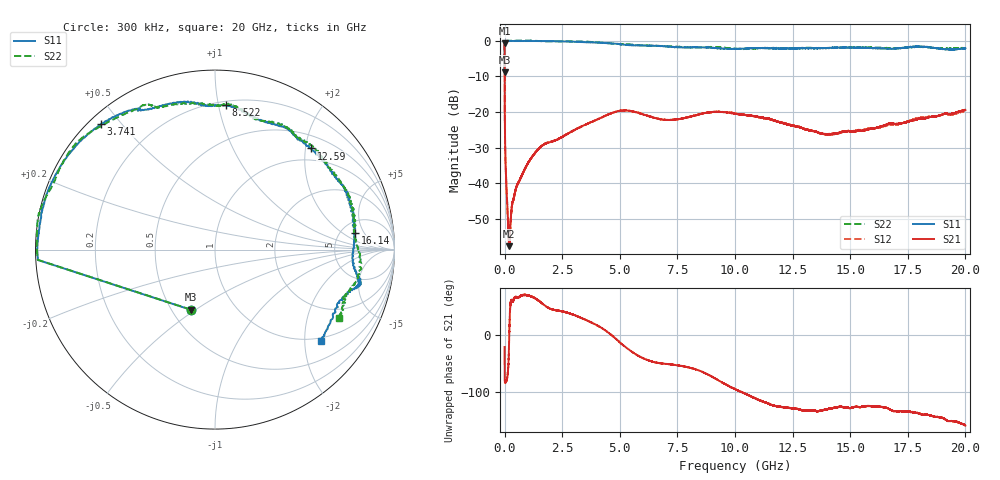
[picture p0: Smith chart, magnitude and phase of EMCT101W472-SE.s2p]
!EMCT101W472
!Johanson Technology Inc.
!www.johansontechnology.com
!Test Board Conditions:
!Substrate Type  RO4350B
!Substrate Thickness  10 mil
!Substrate Dk  3.66
!TL Type: GCPW
!TL Trace Width  22 mil
!TL Gap  14 mil
!PART MODE SINGLE ENDED (AKA BYPASS)
!DUT TOPOLOGY	SERIES-SHUNT
# MHz S  dB  R 50
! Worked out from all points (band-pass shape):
!   20001 points, 300 kHz to 20 GHz, reference 50 ohm
!   highest |S21| = -0.71 dB at 300 kHz (marker M1); lowest = -57.6 dB at 194.3 MHz (marker M2)
!   |S21| within 3 dB of the highest: start of sweep to 872.4 kHz
!   lowest |S11| = -8.8 dB at 300 kHz (marker M3), VSWR 2.13, Z = 31 - j23.9 ohm
!   |S11| at or under -10 dB: nowhere
!   |S22| runs from -8.9 to 0.0 dB; largest |S21 - S12| = 0.0049
!   S11 on the Smith chart (normalised r, x): 300 kHz: 0.62, -0.48; 3.741 GHz: 0.03, +0.44; 8.522 GHz: 0.23, +1.05; 12.59 GHz: 0.74, +2.11; 16.14 GHz: 6.66, +3.26; 20 GHz: 0.90, -2.37
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0.3  -8.84 -112.1  -0.71 -21.6  -0.71 -21.5  -8.86 -112.0
110.298  -0.09 179.1  -45.22 -76.0  -45.23 -75.8  -0.08 179.4
147.298  -0.09 178.5  -50.77 -63.3  -50.48 -64.2  -0.06 178.9
194.297  -0.09 178.0  -57.62 -12.8  -56.81 -13.8  -0.06 178.3
254.296  -0.10 177.4  -51.45 52.7  -51.52 52.6  -0.05 177.4
375.294  -0.11 176.0  -44.68 60.2  -44.68 59.5  -0.05 175.9
531.292  -0.12 174.3  -40.68 64.9  -40.63 64.7  -0.02 174.1
1238.281  -0.11 166.1  -32.15 65.3  -32.19 65.8  -0.04 165.5
1709.274  -0.11 160.6  -29.13 52.1  -29.04 52.5  -0.20 160.2
3334.25  -0.40 137.0  -24.09 29.2  -24.11 29.3  -0.25 141.3
3741.244  -0.49 132.4  -22.90 21.9  -22.91 22.0  -0.39 137.3
5120.223  -1.14 118.1  -19.59 -17.5  -19.63 -17.2  -0.96 115.9
6667.2  -1.50 101.9  -21.94 -49.3  -21.90 -49.7  -1.48 107.4
8522.172  -1.86 85.7  -20.55 -63.7  -20.54 -64.2  -1.93 87.4
10000.15  -2.36 68.4  -20.52 -95.2  -20.38 -95.2  -2.30 75.0
12591.11  -2.20 46.5  -23.96 -129.3  -23.88 -129.1  -2.19 51.4
13334.1  -2.18 35.6  -25.31 -132.2  -25.25 -132.4  -2.07 42.9
16138.06  -2.11 6.9  -24.48 -125.5  -24.44 -127.3  -2.02 11.9
16667.05  -2.29 -1.6  -23.33 -129.3  -23.54 -128.9  -2.11 7.9
18160.03  -1.75 -14.4  -21.75 -139.9  -21.64 -140.1  -1.84 -10.2
19177.01  -2.46 -23.1  -20.38 -149.3  -20.51 -150.9  -2.30 -20.4
20000  -2.15 -41.1  -19.42 -158.6  -19.62 -156.4  -2.06 -28.8
